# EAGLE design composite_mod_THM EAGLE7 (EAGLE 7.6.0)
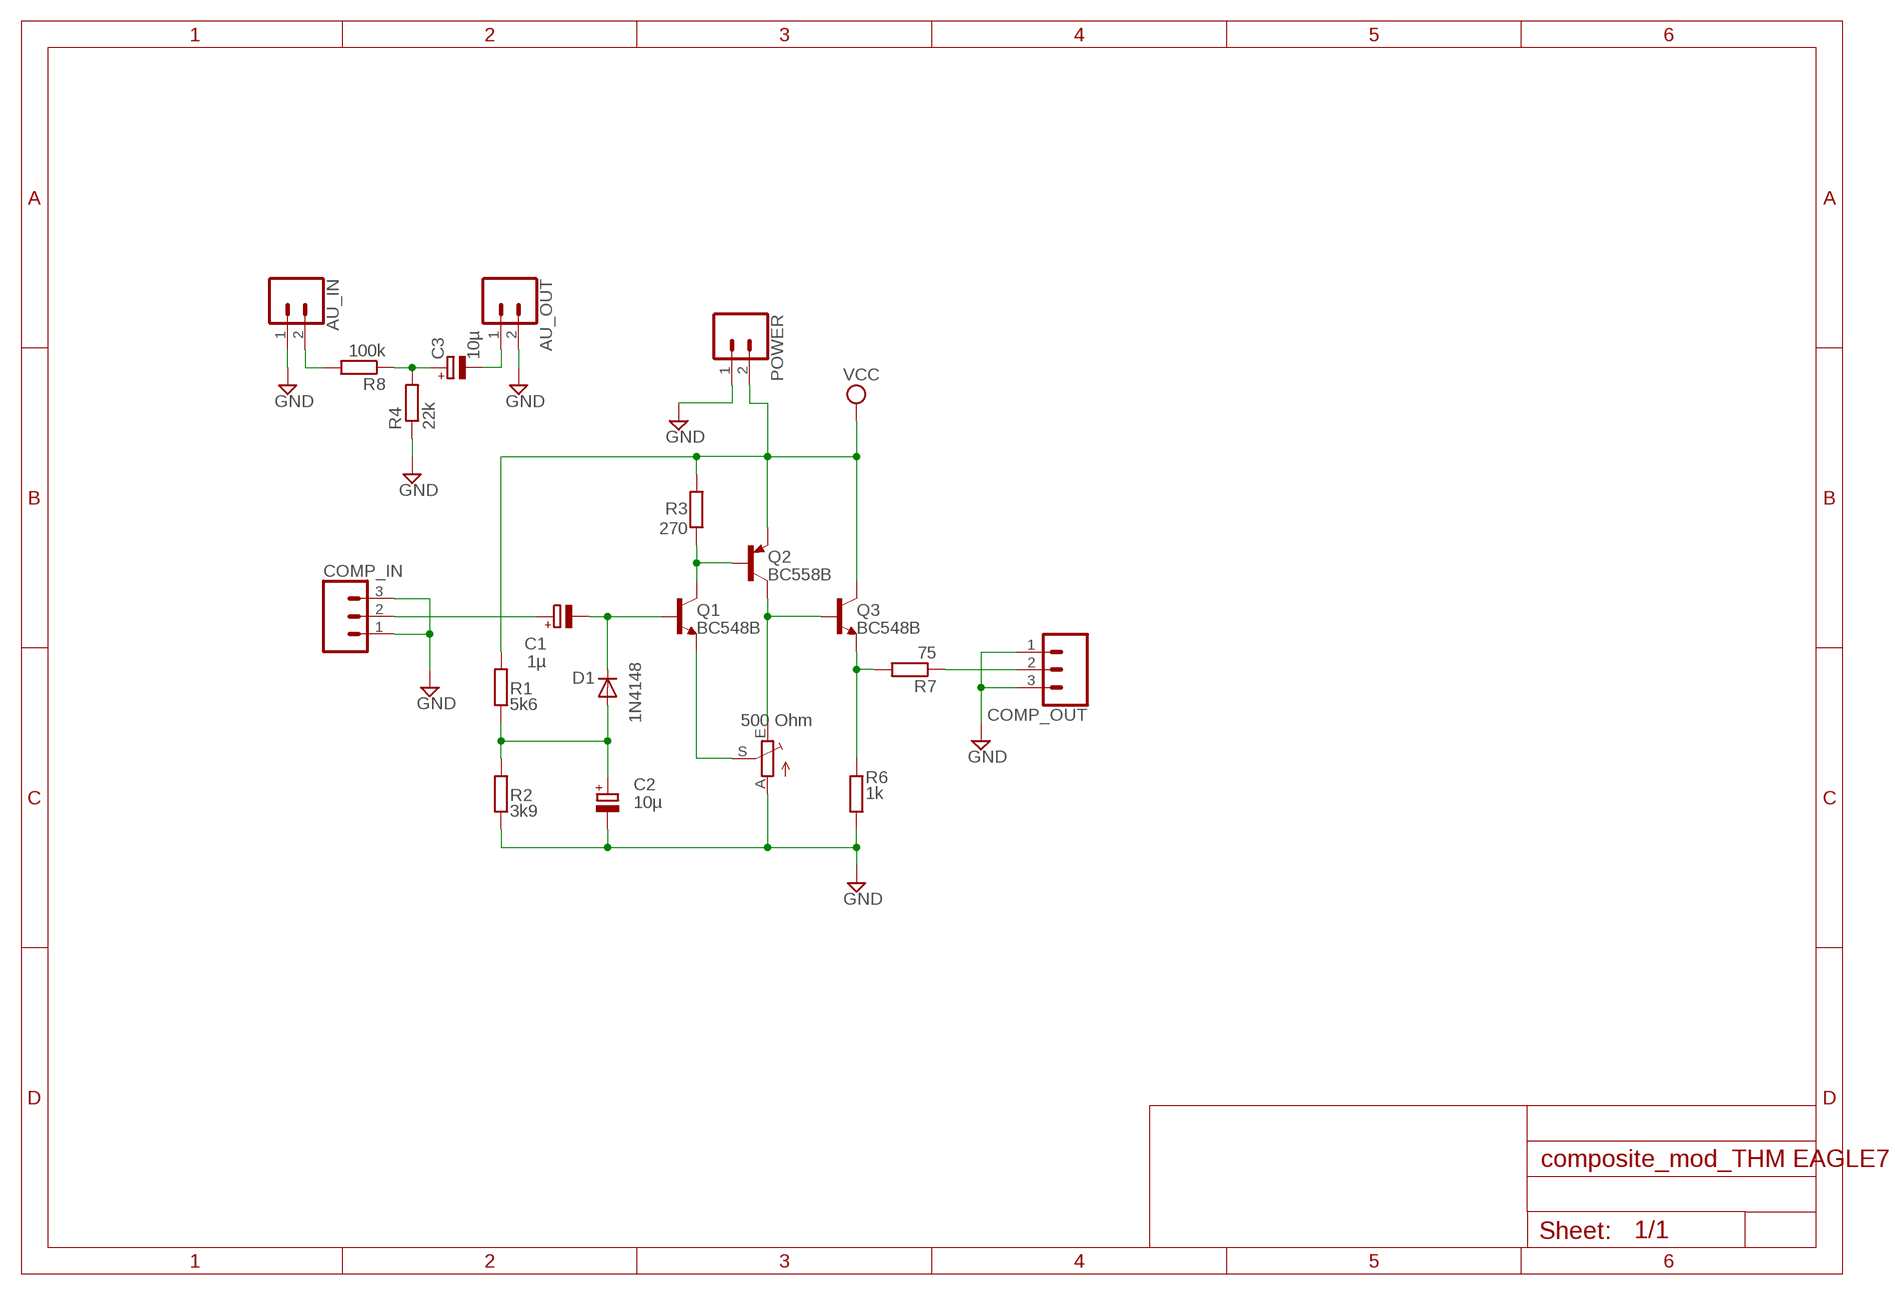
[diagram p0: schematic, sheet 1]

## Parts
AU_IN  CONN_02  [1X02]
AU_OUT  CONN_02  [1X02]
C1  1µ  CPOL-EUE2.5-6  [E2,5-6]
C2  10µ  CPOL-EUE2.5-6  [E2,5-6]
C3  10µ  CPOL-EUE2.5-6  [E2,5-6]
COMP_IN  455-1750-1-ND  CONN_03  [1X03]
COMP_OUT  455-1750-1-ND  CONN_03  [1X03]
D1  1N4148  1N4148DO35-10  [DO35-10]
POT  500 Ohm  TRIM_EU-S64Y  [S64Y]
POWER  CONN_02  [1X02]
Q1  BC548B  [TO92-EBC]
Q2  BC558B  [TO92-EBC]
Q3  BC548B  [TO92-EBC]
R1  5k6  R-EU_0207/10  [0207/10]
R2  3k9  R-EU_0207/10  [0207/10]
R3  270  R-EU_0207/10  [0207/10]
R4  22k  R-EU_0207/10  [0207/10]
R6  1k  R-EU_0207/10  [0207/10]
R7  75  R-EU_0207/10  [0207/10]
R8  100k  R-EU_0207/10  [0207/10]

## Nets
GND: AU_IN.1 AU_OUT.2 C2.- COMP_IN.1 COMP_IN.3 COMP_OUT.1 COMP_OUT.3 POT.A POWER.1 R2.1 R4.1 R6.1
N$2: C3.+ R4.2 R8.1
N$3: AU_IN.2 R8.2
N$4: AU_OUT.1 C3.-
N$5: C2.+ D1.A R1.1 R2.2
N$7: POT.E Q2.C Q3.B
N$10: Q3.E R6.2 R7.2
N$11: COMP_OUT.2 R7.1
N$14: C1.+ COMP_IN.2
VCC [VCC]: POWER.2 Q2.E Q3.C R1.2 R3.2
XE: Q1.C Q2.B R3.1
YB: C1.- D1.C Q1.B
ZC: POT.S Q1.E

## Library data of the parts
AU_IN AU_OUT POWER = SparkFun-Connectors:CONN_02: Multi connection point. Often used as Generic Header-pin footprint for 0.1 inch spaced/style header connections
C1-C3 = rcl:CPOL-EU: POLARIZED CAPACITOR, European symbol
COMP_IN COMP_OUT = SparkFun-Connectors:CONN_03: Multi connection point. Often used as Generic Header-pin footprint for 0.1 inch spaced/style header connections On any of the 0.1 inch spaced packages, you can populate with these: Break Away Headers - Straight (PRT-00116) Break Away Male Headers - Right Angle (PRT-00553) Female Headers (PRT-00115)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; PROD_ID: XXX-00000
D1 = diode:1N4148: DIODE
POT = pot:TRIM_EU-: POTENTIOMETER
Q1 Q3 = transistor-npn:BC548*: NPN Transistor
Q2 = transistor-pnp:BC558*: PNP Transistror
R1-R3 R6 R7 = resistor:R-EU_: RESISTOR, European symbol
R4 R8 = rcl:R-EU_: RESISTOR, European symbol

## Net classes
1 VCC: width 1.016 mm, drill 1 mm, clearance 0.2 mm
2 COUT: width 1.29 mm, drill 1 mm, clearance 2 mm

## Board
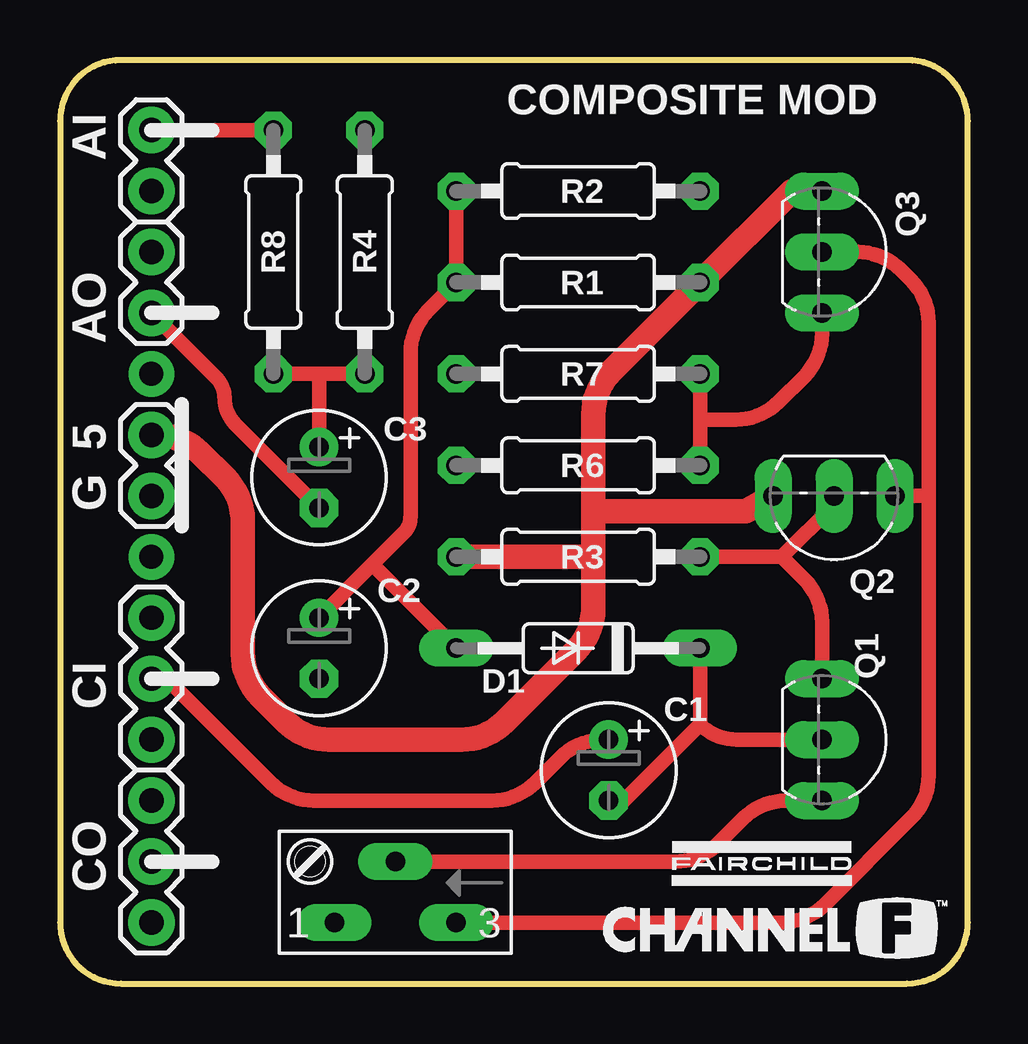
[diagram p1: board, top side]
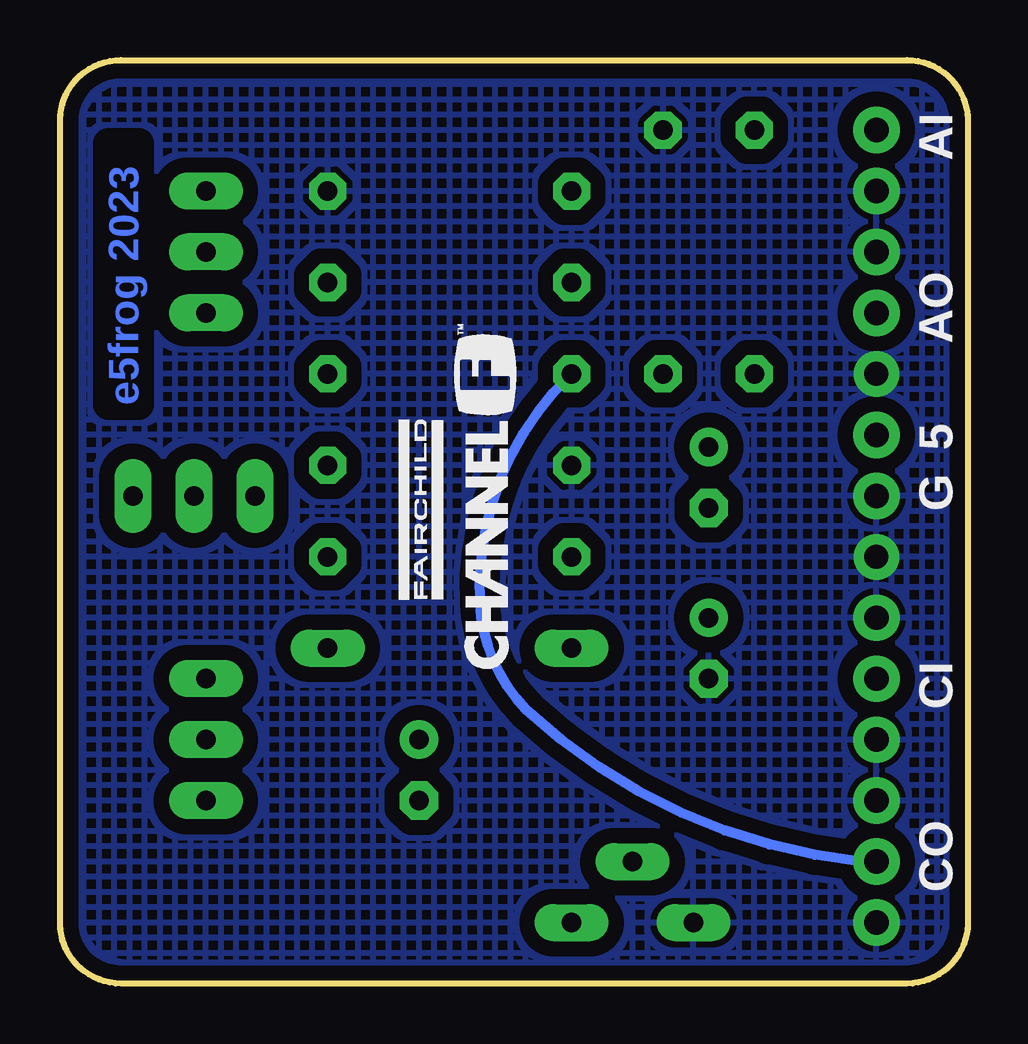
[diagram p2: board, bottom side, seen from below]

Size 37.83 x 38.48 mm. Coordinates in mm from the lower left corner, seen from the top.
Outline: 0,35.94 0,2.54 arc90 2.54,0 35.28,0 arc90 37.83,2.54 37.83,35.94 arc90 35.28,38.48 2.54,38.48 arc90 0,35.94
Copper layers (1*16): Top 0.0356mm / dielectric 1.5011mm / Bottom 0.0356mm
Design rules "Cogra_utvecklarservice *": minimum track width 0.15mm, minimum drill 0.3mm, track to track 0.15mm, track to pad 0.15mm, pad to pad 0.15mm, via to via 0.15mm, smd to smd 0.15mm, copper to edge 10mil, drill to drill 0.5mm, minimum pad ring 0.15mm, minimum via ring 0.15mm, stop-mask expansion 0mil, vias tented up to drill 0mil, thermal gap 10mil

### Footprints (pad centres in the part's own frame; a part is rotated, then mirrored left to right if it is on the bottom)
1X02 = drill 1.016 pad 1.88: 1 0,0; 2 2.54,0
E2,5-6 = drill 0.813 pad 1.6: + -1.27,0 | drill 0.813 pad 1.6 octagon: - 1.27,0
1X03 = drill 1.016 pad 1.88: 1 0,0; 2 2.54,0; 3 5.08,0
DO35-10 = drill 0.813 long: A 5.08,0; C -5.08,0
S64Y = drill 0.813 long: A 2.54,1.27; E -2.54,1.27; S 0,-1.27
TO92-EBC = drill 0.813 long: B 0,-1.27; C -2.54,-1.27; E 2.54,-1.27
0207/10 = drill 0.813 octagon: 1 -5.08,0; 2 5.08,0

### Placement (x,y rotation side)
AU_IN  3.81,33.02 90 top
AU_OUT  3.81,27.94 90 top
C1  22.86,8.89 270 top
C2  10.79,13.97 270 top
C3  10.79,21.08 270 top
COMP_IN  3.81,15.24 270 top
COMP_OUT  3.81,7.62 270 top
D1  21.59,13.97 180 top
POT  13.97,3.81 180 top
POWER  3.81,20.32 90 top
Q1  33.02,10.16 270 top
Q2  32.25,19.05 180 top
Q3  33.02,30.48 270 top
R1  21.59,29.21 0 top
R2  21.59,33.02 180 top
R3  21.59,17.78 180 top
R4  12.7,30.48 270 top
R6  21.59,21.59 0 top
R7  21.59,25.4 0 top
R8  8.89,30.48 90 top

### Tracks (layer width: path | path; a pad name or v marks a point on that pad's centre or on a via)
GND  (via drill 1)
  other vias: 3.81,17.78 3.81,25.4
  pour Bottom (isolate 0.635, hatched): -0.64,38.73 -0.64,0 38.73,0 38.73,38.73
N$2
  Top 0.61: R8.1 10.79,25.4 | 10.79,25.4 R4.2 | C3.+ 10.79,25.4
N$3
  Top 0.61: AU_IN.2 R8.2
N$4
  Top 0.61: AU_OUT.1 6.5,25.25 arc-45 6.86,24.38 arc45 7.31,23.3 C3.-
N$5
  Top 0.61: R2.2 R1.1 15.35,28.05 arc45 14.61,26.25 14.61,19.47 arc-45 14.31,18.75 12.95,17.4 | C2.+ 12.95,17.4 | D1.A 13.17,17.31 arc45 12.95,17.4
N$7
  Top 0.61: POT.E 30.06,2.54 arc45 31.86,3.28 35.45,6.88 arc45 36.2,8.67 36.2,20.32 | 36.2,20.32 36.2,27.52 arc45 35.45,29.32 35.03,29.74 arc45 33.24,30.48 Q3.B | Q2.C 36.2,20.32
N$10
  Top 0.61: R6.2 26.67,23.5 | 26.67,23.5 R7.2 | Q3.E 31.75,27.09 arc-45 31.01,25.29 29.95,24.24 arc-45 28.16,23.5 26.67,23.5
N$11
  Bottom 0.406: COMP_OUT.2 4.45,5.08 arc37 18.41,11.43 arc41 20.32,15.88 arc49 R7.1
N$14
  Top 0.61: C1.+ 22.64,10.16 arc45 20.85,9.42 19.79,8.36 arc-45 18,7.62 10.58,7.62 arc-45 8.78,8.36 4.89,12.25 arc45 COMP_IN.2
VCC
  Top 1.016: POWER.2 4.03,22.86 arc-45 5.82,22.12 6.88,21.06 arc-45 7.62,19.27 7.62,13.75 arc45 8.36,11.96 9.42,10.9 arc45 11.21,10.16 16.73,10.16 arc45 18.52,10.9 21.48,13.86 arc45 22.23,15.66 22.23,17.78 | 22.23,17.78 22.23,19.68 | 22.23,19.68 22.23,23.71 arc-45 22.97,25.51 R1.2 30.48,33.02 Q3.C | R3.2 22.23,17.78 | 22.23,19.68 28.57,19.68 Q2.E
XE
  Top 0.61: R3.1 30.08,17.78 | 30.08,17.78 32.25,19.95 Q2.B | Q1.C 31.75,15.06 arc45 31.01,16.85 30.08,17.78
YB
  Top 0.61: D1.C 26.67,10.79 | C1.- 23.5,7.62 26.67,10.79 | 26.67,10.79 arc45 28.2,10.16 Q1.B
ZC
  Top 0.61: POT.S 25.62,5.08 arc45 27.41,5.82 28.47,6.88 arc-45 30.26,7.62 Q1.E

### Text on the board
Bottom: e5frog 2023
tPlace: COMPOSITE MOD | AI | AO | 5 | G | CI | CO
bPlace: AI | AO | 5 | G | CI | CO
bStop: e5frog 2023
